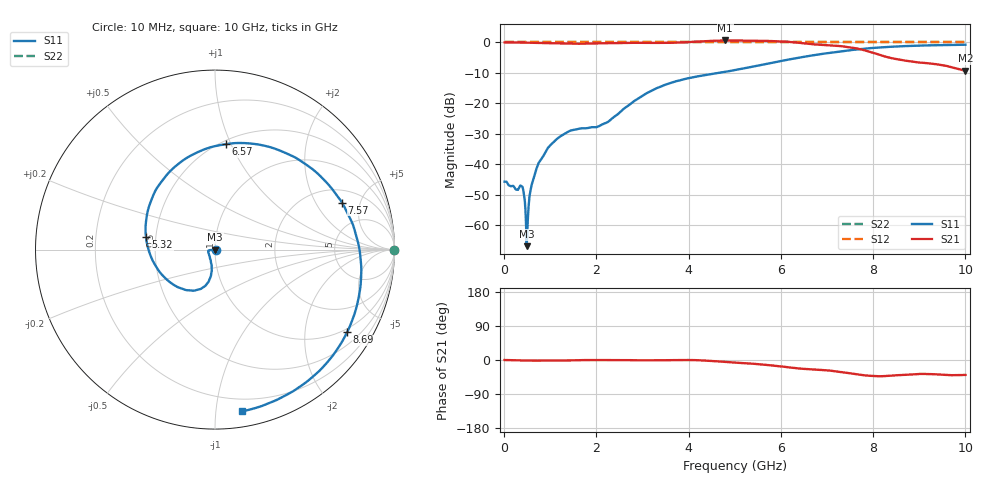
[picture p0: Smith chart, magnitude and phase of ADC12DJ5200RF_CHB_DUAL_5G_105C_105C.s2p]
! Texas Instruments, Inc.
! ADC12DJ5200RF - CH B S-Parameters (Dual Ch Mode, Fs = 5 GSPS, 105 degC case, 105 degC juntion)
! Port 1 represents the 100-ohm differenal input, Port 2 the digital output
! freq  dbS11  angS11  dbS21 angS21 dbS12 angS12 dbS22 angS22
# HZ S DB R 100
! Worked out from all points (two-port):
!   1000 points, 10 MHz to 10 GHz, reference 100 ohm
!   highest |S21| = 0.62 dB at 4.79 GHz (marker M1); lowest = -9.3 dB at 10 GHz (marker M2)
!   |S21| within 3 dB of the highest: start of sweep to 7.757 GHz
!   lowest |S11| = -66.8 dB at 490 MHz (marker M3), VSWR 1.00, Z = 100 + j0.0909 ohm
!   |S11| at or under -10 dB: start of sweep to 4.655 GHz
!   |S22| runs from 0.0 to 0.0 dB; largest |S21 - S12| = 0.77
!   S11 on the Smith chart (normalised r, x): 10 MHz: 1.01, -0.00; 5.32 GHz: 0.44, +0.07; 6.57 GHz: 0.53, +0.96; 7.57 GHz: 2.79, +3.39; 8.69 GHz: 0.87, -3.26; 10 GHz: 0.11, -1.18
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1e7  -45.69 -2.8  0.00 -0.0  0.00 0.0  0.00 0.0
3.8e8  -47.17 -16.4  -0.05 -1.2  0.00 0.0  0.00 0.0
4.9e8  -66.84 93.5  -0.09 -1.5  0.00 0.0  0.00 0.0
5.2e8  -56.15 -177.4  -0.10 -1.5  0.00 0.0  0.00 0.0
5.8e8  -47.93 -158.5  -0.12 -1.6  0.00 0.0  0.00 0.0
6.5e8  -44.16 -162.0  -0.17 -1.7  0.00 0.0  0.00 0.0
9.2e8  -35.36 -172.3  -0.25 -1.7  0.00 0.0  0.00 0.0
1.25e9  -30.53 -174.5  -0.39 -1.5  0.00 0.0  0.00 0.0
1.68e9  -28.19 -167.0  -0.43 -0.3  0.00 0.0  0.00 0.0
2.22e9  -26.31 -127.8  -0.24 -0.2  0.00 0.0  0.00 0.0
3.34e9  -14.84 -101.2  -0.18 -0.8  0.00 0.0  0.00 0.0
4.79e9  -9.65 -156.0  0.62 -5.1  0.00 0.0  0.00 0.0
5.01e9  -9.07 -169.7  0.61 -7.0  0.00 0.0  0.00 0.0
5.32e9  -8.17 169.9  0.53 -9.3  0.00 0.0  0.00 0.0
5.9e9  -6.42 130.4  0.37 -15.7  0.00 0.0  0.00 0.0
6.57e9  -4.57 84.1  -0.41 -23.9  0.00 0.0  0.00 0.0
6.67e9  -4.31 77.3  -0.58 -24.8  0.00 0.0  0.00 0.0
7.09e9  -3.36 49.3  -0.98 -28.4  0.00 0.0  0.00 0.0
7.57e9  -2.45 20.4  -1.81 -36.2  0.00 0.0  0.00 0.0
8.34e9  -1.48 -18.1  -4.97 -41.8  0.00 0.0  0.00 0.0
8.69e9  -1.23 -32.1  -5.98 -39.1  0.00 0.0  0.00 0.0
1e10  -0.78 -80.5  -9.32 -39.5  0.00 0.0  0.00 0.0
